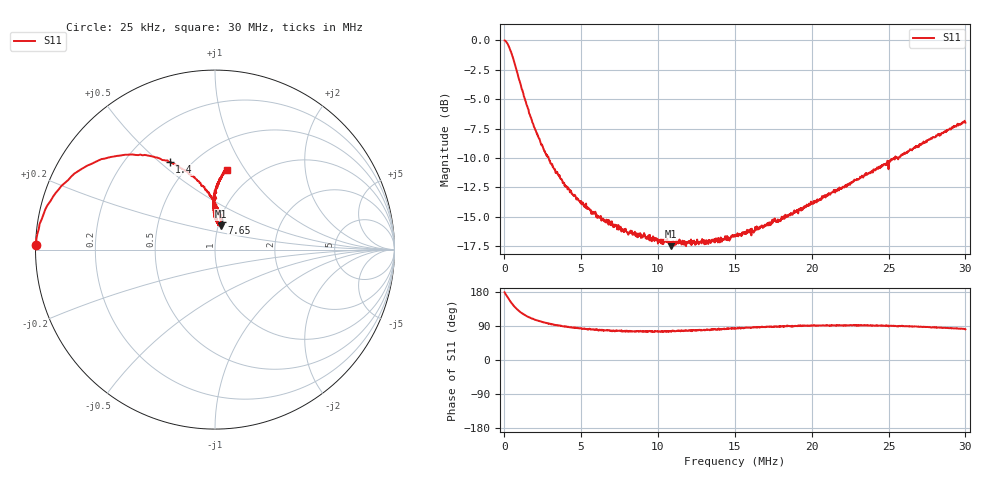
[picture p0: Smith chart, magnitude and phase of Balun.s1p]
! Touchstone file generated by AntScope (RigExpert AA-54 antenna analyzer)
# MHz Z RI R 50
! Format: Frequency Z-real Z-imaginary (normalized to 50 Ohm)
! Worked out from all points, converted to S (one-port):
!   1200 points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, 25 kHz to 30 MHz, reference 50 ohm
!   lowest |S11| = -17.5 dB at 10.85 MHz (marker M1), VSWR 1.31, Z = 51.4 + j13.6 ohm
!   |S11| at or under -10 dB: 2.89 MHz to 25.32 MHz (22.43 MHz wide, 159 % of centre); 25.32724 MHz to 25.36687 MHz (39.63 kHz wide, 0.156 % of centre); 25.37862 MHz to 25.41492 MHz (36.3 kHz wide, 0.143 % of centre)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
!   S11 on the Smith chart (normalised r, x): 25 kHz: 0.00, +0.01; 1.4 MHz: 0.39, +0.54; 7.65 MHz: 1.03, +0.32; 30 MHz: 0.75, +0.83
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0.025  0.001 0.0124
0.1  0.0058 0.0584
0.2  0.0146 0.1172
0.375  0.0462 0.2116
0.5  0.0744 0.2748
0.625  0.1106 0.3326
0.775  0.1602 0.391
1  0.2388 0.4632
1.2  0.3138 0.5094
1.4  0.3856 0.5396
1.75  0.5054 0.5668
2.2  0.632 0.5716
2.9  0.775 0.5372
3.775  0.8844 0.4798
4.55  0.9398 0.429
5.625  0.992 0.3824
7.525  1.019 0.323
7.65  1.032 0.3206
10.15  1.036 0.2878
10.85  1.028 0.272
11.275  1.025 0.2848
13.125  1.012 0.2766
15.025  0.994 0.2956
16.15  0.9728 0.3068
18.775  0.9362 0.3538
22.525  0.8678 0.4544
26.275  0.8042 0.6134
30  0.7538 0.8318
